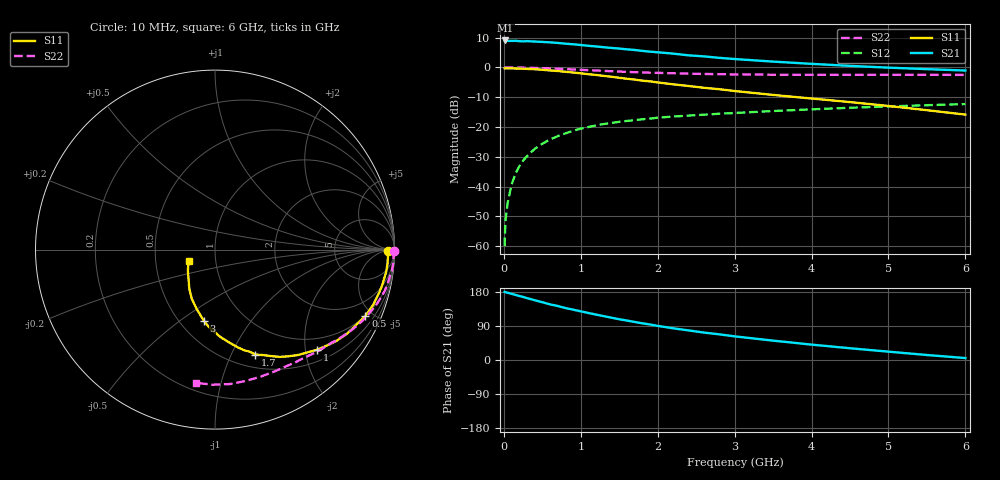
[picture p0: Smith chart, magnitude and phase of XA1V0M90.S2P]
! SIEMENS Discrete & RF Semiconductors
! BFY180
! Si NPN RF Bipolar Junction Transistor in MICRO-X
! VCE = 1 V  IC = 0.9 mA
! Common Emitter S-Parameters:  May  1997
# GHz  S  MA  R  50
!  f  S11  S21  S12  S22
! GHz  MAG  ANG  MAG  ANG  MAG  ANG  MAG  ANG
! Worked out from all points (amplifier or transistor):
!   36 points, 10 MHz to 6 GHz, reference 50 ohm
!   highest |S21| = 9.1 dB at 20 MHz (marker M1)
!   |S21| within 3 dB of that: start of sweep to 1.611 GHz
!   unconditionally stable (mu >= 1): 3.283 GHz to end of sweep
!   at 250 MHz: K = 0.08, MSG = 20.0 dB, |S12| = -31.3 dB
!   at 1.4 GHz: K = 0.56, MSG = 12.6 dB, |S12| = -18.6 dB
!   at 6 GHz: K = 1.11, MAG = 3.6 dB, |S12| = -12.3 dB
!   S11 on the Smith chart (normalised r, x): 10 MHz: 55, -8; 500 MHz: 0.99, -4.54; 1 GHz: 0.74, -2.25; 1.7 GHz: 0.64, -1.24; 3 GHz: 0.65, -0.62; 6 GHz: 0.74, -0.10
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0.01  0.9647 -0.3  2.77 179.7  0.001 82.4  0.997 -0.3
0.02  0.9638 -0.8  2.84 178.8  0.0026 92.3  0.9999 -0.6
0.05  0.9641 -2.4  2.795 177.4  0.0054 86.7  0.9958 -1.4
0.1  0.9644 -4.6  2.79 174.7  0.0107 87.8  0.9961 -2.8
0.15  0.9618 -7.5  2.801 171.9  0.0163 85.2  0.9956 -4.2
0.25  0.952 -12.2  2.74 166.5  0.0273 82.2  0.9931 -7.0
0.3  0.9465 -14.4  2.768 163.3  0.0323 80.1  0.9866 -8.3
0.5  0.9158 -23.8  2.682 152.4  0.0523 73.3  0.9728 -13.7
0.6  0.8913 -28.1  2.638 146.8  0.0618 70.3  0.9624 -16.2
0.8  0.8463 -37.0  2.508 137.1  0.0783 63.9  0.9368 -21.1
1  0.7976 -44.3  2.384 128.4  0.0938 58.5  0.9131 -25.6
1.1  0.7706 -48.0  2.308 124.0  0.1 56.3  0.9005 -27.5
1.4  0.6973 -59.0  2.126 111.5  0.1173 49.7  0.8639 -33.5
1.7  0.6267 -68.9  1.966 100.4  0.1304 44.7  0.8316 -38.5
2  0.56 -76.8  1.798 90.0  0.1435 40.5  0.8119 -43.2
2.2  0.5212 -81.6  1.708 83.7  0.1498 37.6  0.7985 -46.2
2.6  0.456 -90.8  1.535 72.4  0.1611 33.4  0.7773 -51.7
3  0.4025 -98.8  1.385 62.4  0.172 29.5  0.7646 -57.0
3.5  0.3458 -107.2  1.254 51.1  0.1857 25.5  0.756 -63.5
4.5  0.2623 -123.0  1.063 31.0  0.2106 17.2  0.7516 -76.9
5.5  0.1917 -142.0  0.937 13.2  0.2326 9.0  0.7529 -90.9
6  0.1616 -155.9  0.888 5.1  0.2428 4.6  0.7499 -98.0
